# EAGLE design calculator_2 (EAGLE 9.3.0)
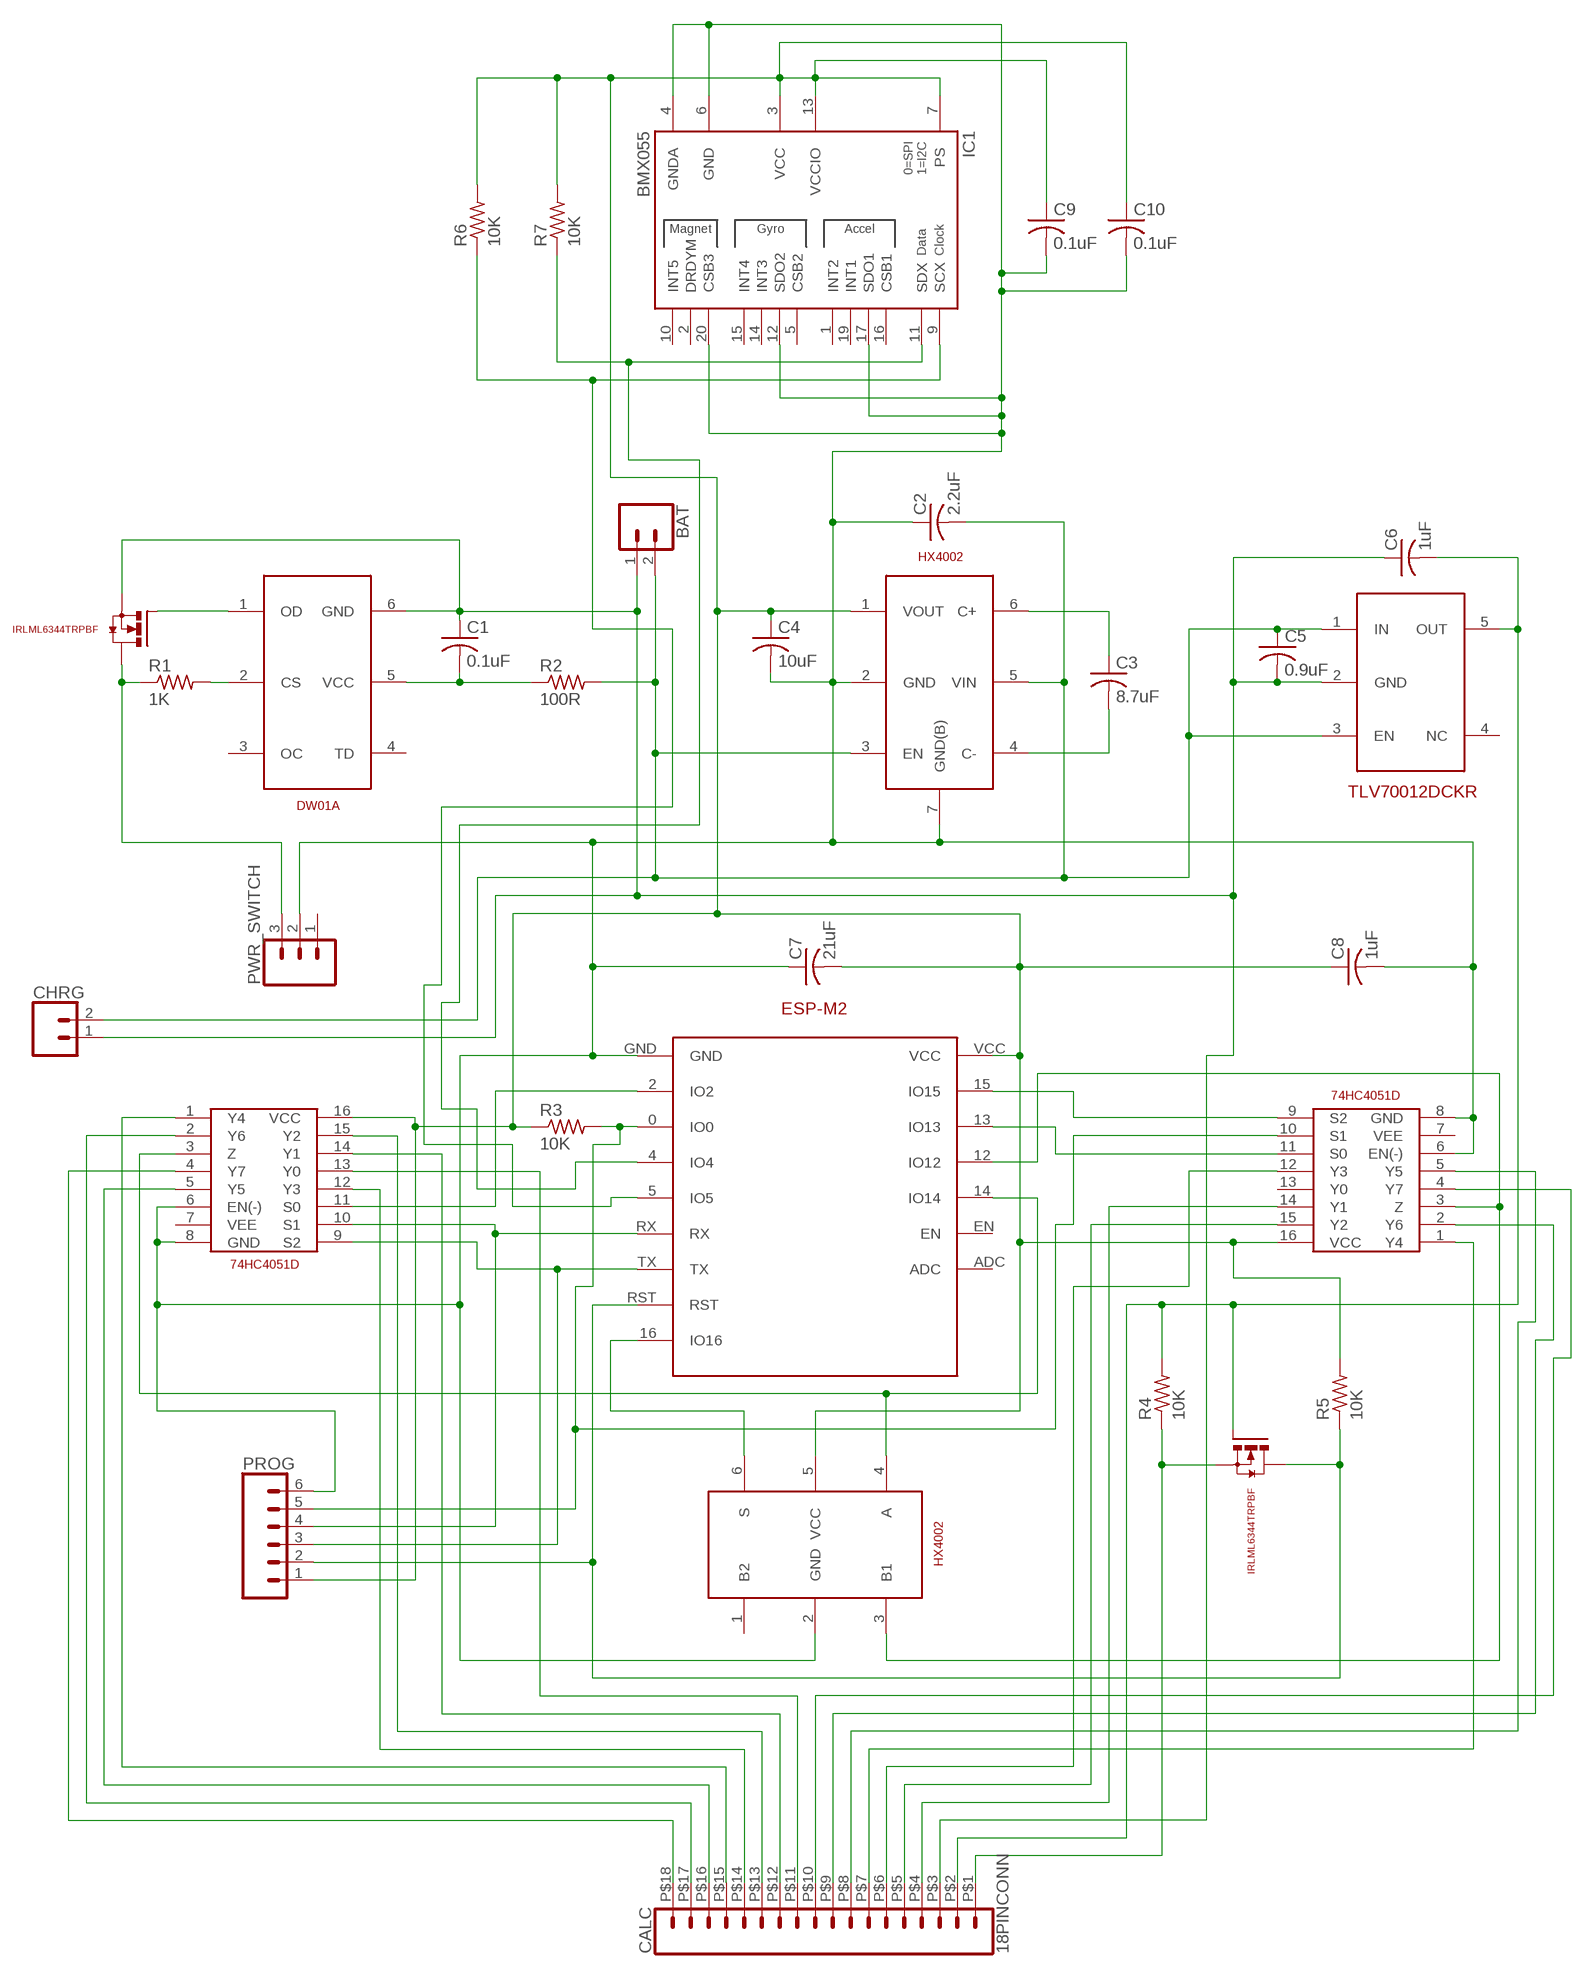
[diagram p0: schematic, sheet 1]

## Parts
BAT  CONN_021X02_NO_SILK  [1X02_NO_SILK]
C1  0.1uF  C-USC0402  [C0402]
C2  2.2uF  C-USC0603  [C0603]
C3  8.7uF  C-USC0402  [C0402]
C4  10uF  C-USC0402  [C0402]
C5  0.9uF  C-USC0402  [C0402]
C6  1uF  C-USC0402  [C0402]
C7  21uF  C-USC0603  [C0603]
C8  1uF  C-USC0603  [C0603]
C9  0.1uF  C-USC0402  [C0402]
C10  0.1uF  C-USC0402  [C0402]
CALC  18PINCONN  [18PINCONN]
CHRG  CONN_021X02_NO_SILK  [1X02_NO_SILK]
ESP-M2  ESP-M2  [ESP-M2]
IC1  BMX055  [BMX055]
IRLML6344  IRLML6344TRPBF6344TRPBF  [SOT-23-3]
PROG  CONN_06NO_SILK_FEMALE_PTH  [1X06_NO_SILK]
PWR_SWITCH  CONN_031X03_NO_SILK  [1X03_NO_SILK]
R1  1K  R-US_R0402  [R0402]
R2  100R  R-US_R0402  [R0402]
R3  10K  R-US_R0402  [R0402]
R4  10K  R-US_R0402  [R0402]
R5  10K  R-US_R0402  [R0402]
R6  10K  R-US_R0402  [R0402]
R7  10K  R-US_R0402  [R0402]
U2  74HC4051  [SOIC-16]
U3  74HC4051  [SOIC-16]
U4  IRLML6344TRPBF6344TRPBF  [SOT-23-3]
U$2  DW01A  [SOT-23-6]
U$3  HX4002  [SOT-23-6(BOTTOM)]
U$4  TLV70012DCKR  [SC70-5]
U$6  SN74LVC1G3157DBVR  [SOT-23-6]

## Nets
GND: C2.1 C4.2 C7.1 C8.2 C9.2 C10.2 ESP-M2.GND IC1.4(GNDA) IC1.6(GND) IC1.12(SDO2) IC1.17(SDO1) IC1.20(CSB3) PROG.6 PWR_SWITCH.2 U2.6(EN(-)) U2.8(GND) U3.6(EN(-)) U3.8(GND) U$3.2(GND) U$3.7(GND(B)) U$6.2(GND)
N$1: IRLML6344.1(G) U$2.1(OD)
N$2: C4.1 C7.2 C8.1 C9.1 C10.1 ESP-M2.VCC IC1.3(VCC) IC1.7(PS) IC1.13(VCCIO) PROG.1 R3.1 R5.2 R6.2 R7.2 U2.16(VCC) U3.16(VCC) U$3.1(VOUT) U$6.5(VCC)
N$3: R1.2 U$2.2(CS)
N$4: BAT.2 C2.2 C5.1 CHRG.2 R2.2 U$3.3(EN) U$3.5(VIN) U$4.1(IN) U$4.3(EN)
N$5: C1.2 R2.1 U$2.5(VCC)
N$6: ESP-M2.0(IO0) PROG.5 R3.2 U3.10(S1)
N$7: C3.1 U$3.6(C+)
N$8: C3.2 U$3.4(C-)
N$9: ESP-M2.13(IO13) U3.11(S0)
N$10: BAT.1 C1.1 C5.2 C6.1 CALC.P$3 CHRG.1 IRLML6344.2(S) U$2.6(GND) U$4.2(GND)
N$11: C6.2 CALC.P$2 R4.2 U4.1(G) U$4.5(OUT)
N$12: ESP-M2.14(IO14) U2.3(Z) U$6.4(A)
N$13: ESP-M2.15(IO15) U3.9(S2)
N$14: ESP-M2.12(IO12) U3.3(Z) U$6.3(B1)
N$15: ESP-M2.TX PROG.3 U2.9(S2)
N$16: ESP-M2.2(IO2) U2.11(S0)
N$17: ESP-M2.RX PROG.4 U2.10(S1)
N$18: ESP-M2.16(IO16) U$6.6(S)
N$19: CALC.P$1 R4.1 U4.2(S)
N$20: IRLML6344.3(D) PWR_SWITCH.3 R1.1
N$21: ESP-M2.4(IO4) IC1.11(SDX) R7.1
N$22: ESP-M2.RST PROG.2 R5.1 U4.3(D)
N$23: CALC.P$4 U3.14(Y1)
N$24: CALC.P$5 U3.15(Y2)
N$25: CALC.P$6 U3.12(Y3)
N$26: CALC.P$7 U3.1(Y4)
N$27: CALC.P$8 U3.5(Y5)
N$28: CALC.P$9 U3.2(Y6)
N$29: CALC.P$10 U3.4(Y7)
N$30: CALC.P$11 U2.13(Y0)
N$31: CALC.P$12 U2.14(Y1)
N$32: CALC.P$13 U2.15(Y2)
N$33: CALC.P$14 U2.12(Y3)
N$34: CALC.P$15 U2.1(Y4)
N$35: CALC.P$16 U2.5(Y5)
N$36: CALC.P$17 U2.2(Y6)
N$37: CALC.P$18 U2.4(Y7)
N$41: ESP-M2.5(IO5) IC1.9(SCX) R6.1
Unconnected: ESP-M2.ADC ESP-M2.EN IC1.1(INT2) IC1.2(DRDYM) IC1.5(CSB2) IC1.10(INT5) IC1.14(INT3) IC1.15(INT4) IC1.16(CSB1) IC1.19(INT1) PWR_SWITCH.1 U2.7(VEE) U3.7(VEE) U3.13(Y0) U$2.3(OC) U$2.4(TD) U$4.4(NC) U$6.1(B2)

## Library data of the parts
BAT CHRG = wifi-calculator-lib:CONN_02: Multi connection point. Often used as Generic Header-pin footprint for 0.1 inch spaced/style header connections
C1-C10 = wifi-calculator-lib:C-US: CAPACITOR, American symbol
CALC = wifi-calculator-lib:18PINCONN
ESP-M2 = wifi-calculator-lib:ESP-M2: ESP8285 Module - M2
IC1 = wifi-calculator-lib:BMX055: Bosch BMX055 Absolute Orientation Sensor (Accelerometer, Gyroscope, Magnetometer)
IRLML6344 U4 = wifi-calculator-lib:IRLML6344TRPBF: N-Channel MOSFET HEXFET® Documentation Datasheet; CATEGORY: Discrete Semiconductor Products; CURRENT-CONTINUOUS_DRAIN: 5A (Ta); DESCRIPTION: MOSFET N-CH 30V 5A SOT23; DOCUMENTATION_LINK: <a href="http://www.irf.com/product-info/datasheets/data/irlml6344pbf.pdf">Datasheet</a>; DOCUMENTATION_URL: http://www.irf.com/product-info/datasheets/data/irlml6344pbf.pdf; DRAIN_TO_SOURCE_VOLTAGE: 30V; FAMILY: FETs - Single; FET_FEATURE: Logic Level Gate; FET_TYPE: MOSFET N-Channel, Metal Oxide; GATE_CHARGE: 6.8nC @ 4.5V; INPUT_CAPACITANCE: 650pF @ 25V; MANUFACTURER: International Rectifier; MOUNTING_TYPE: Surface Mount; PACKAGE: TO-236-3, SC-59, SOT-23-3; PART_NUMBER: IRLML6344TRPBF; POWER-MAX: 1.3W; RDS_ON: 29 mOhm @ 5A, 4.5V; SERIES: HEXFET; SUPPLIER_DEVICE_PACKAGE: SOT-23; SUPPLIER_ITEM_LINK: <a href="http://www.digikey.com/product-detail/en/IRLML6344TRPBF/IRLML6344TRPBFCT-ND/2538168">Details</a>; SUPPLIER_ITEM_NUMBER: IRLML6344TRPBFCT-ND; SUPPLIER_ITEM_URL: http://www.digikey.com/product-detail/en/IRLML6344TRPBF/IRLML6344TRPBFCT-ND/2538168; SUPPLIER_LINK: <a href="http://www.digikey.com">Home Page</a>; SUPPLIER_NAME: Digi-Key; SUPPLIER_URL: http://www.digikey.com; VGS: 1.1V @ 10uA
PROG = wifi-calculator-lib:CONN_06: Multi connection point. Often used as Generic Header-pin footprint for 0.1 inch spaced/style header connections On any of the 0.1 inch spaced packages, you can populate with these: Break Away Headers - Straight (PRT-00116) Break Away Male Headers - Right Angle (PRT-00553) Female Headers (PRT-00115)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; PROD_ID: CONN-08437
PWR_SWITCH = wifi-calculator-lib:CONN_03: Multi connection point. Often used as Generic Header-pin footprint for 0.1 inch spaced/style header connections On any of the 0.1 inch spaced packages, you can populate with these: Break Away Headers - Straight (PRT-00116) Break Away Male Headers - Right Angle (PRT-00553) Female Headers (PRT-00115)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
R1-R7 = wifi-calculator-lib:R-US_: RESISTOR, American symbol
U2 U3 = wifi-calculator-lib:74HC4051: 8 Channel Analog Multiplexer/Demultiplexer
U$2 = wifi-calculator-lib:DW01A: Lithium battery protection IC
U$3 = wifi-calculator-lib:HX4002: 3.3V Output, Buck & Boost Converter
U$4 = wifi-calculator-lib:TLV70012DCKR: 1.2V LDO Voltage Regulator
U$6 = wifi-calculator-lib:SN74LVC1G3157DBVR: Single-Pole Double-Throw Analog Switch

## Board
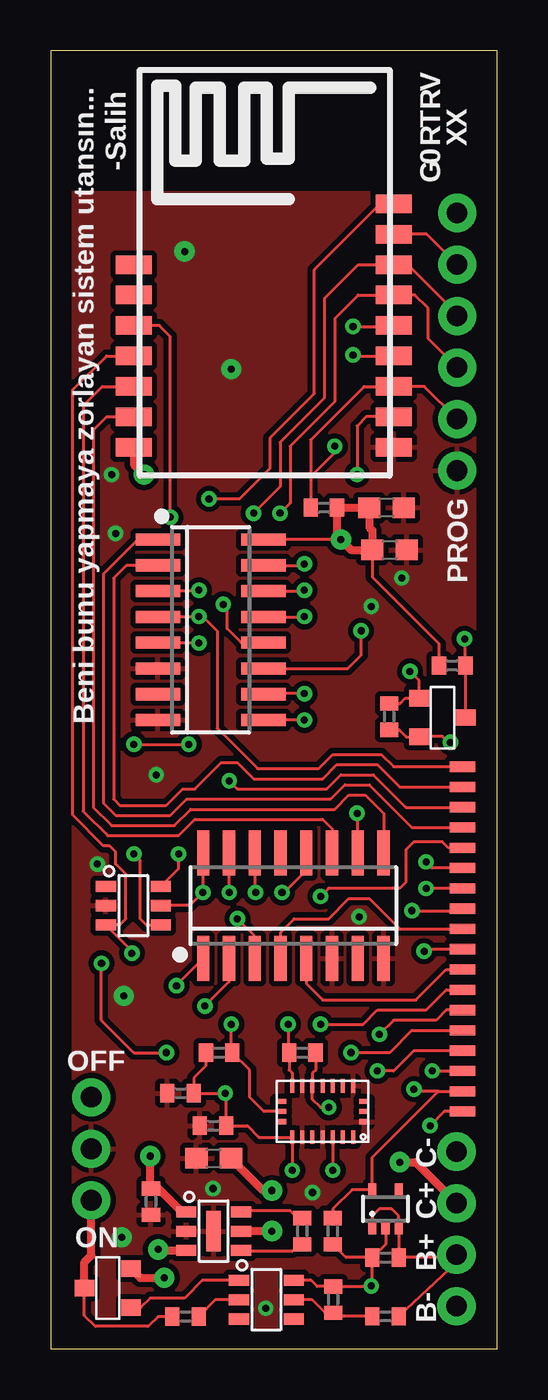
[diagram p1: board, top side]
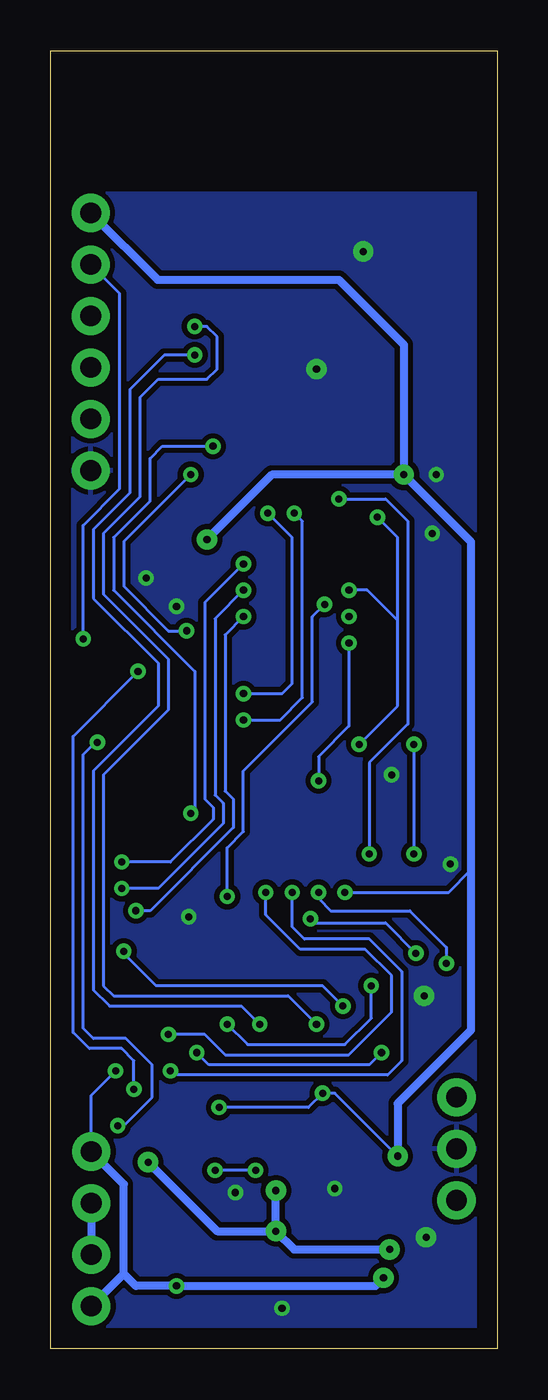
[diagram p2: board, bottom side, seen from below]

Size 22 x 64 mm. Coordinates in mm from the lower left corner, seen from the top.
Outline: 0,0 22,0 22,64 0,64 0,0
Copper layers (1*16): Top 0.035mm / dielectric 1.5mm / Bottom 0.035mm
Design rules "default *": minimum track width 6mil, minimum drill 0.35mm, track to track 6mil, track to pad 6mil, pad to pad 6mil, via to via 6mil, smd to smd 6mil, copper to edge 40mil, drill to drill 6mil, minimum pad ring 10mil, minimum via ring 8mil, stop-mask expansion 4mil, vias tented up to drill 14mil, thermal gap 10mil

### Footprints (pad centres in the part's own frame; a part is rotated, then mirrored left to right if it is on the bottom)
1X02_NO_SILK = drill 1.016 pad 1.88: 1 0,0; 2 2.54,0
C0402 = smd 0.7 x 0.9: 1 -0.65,0; 2 0.65,0
C0603 = smd 1.1 x 1: 1 -0.85,0; 2 0.85,0
18PINCONN = smd 0.5 x 1.27: P$1 -8.5,0; P$2 -7.5,0; P$3 -6.5,0; P$4 -5.5,0; P$5 -4.5,0; P$6 -3.5,0; P$7 -2.5,0; P$8 -1.5,0; P$9 -0.5,0; P$10 0.5,0; P$11 1.5,0; P$12 2.5,0; P$13 3.5,0; P$14 4.5,0; P$15 5.5,0; P$16 6.5,0; P$17 7.5,0; P$18 8.5,0
ESP-M2 = smd 1.778 x 0.914: 0 6,-6.4; 2 6,-7.9; 4 6,-4.9; 5 6,-3.4; 12 -6.8,-4.9; 13 -6.8,-6.4; 14 -6.8,-3.4; 15 -6.8,-7.9; 16 6,2.599; ADC -6.8,-0.4; EN -6.8,-1.9; GND 6,-9.4; RST 6,1.1; RX 6,-1.9; TX 6,-0.4; VCC -6.8,-9.4
BMX055 = smd 0.25 x 0.675: 1 -1.5,1.262; 2 -1,1.262; 3 -0.5,1.262; 4 0,1.262; 5 0.5,1.262; 6 1,1.262; 7 1.5,1.262; 11 1.5,-1.262; 12 1,-1.262; 13 0.5,-1.262; 14 0,-1.262; 15 -0.5,-1.262; 16 -1,-1.262; 17 -1.5,-1.262 | smd 0.55 x 0.25: 8 2.05,0.5; 9 2.05,0; 10 2.05,-0.5; 18 -2.05,-0.5; 19 -2.05,0; 20 -2.05,0.5
SOT-23-3 = smd 0.802 x 0.972: 1 -0.96,-1.15; 2 0.95,-1.15; 3 0,1.15
1X06_NO_SILK = drill 1.016 pad 1.88: 1 0,0; 2 2.54,0; 3 5.08,0; 4 7.62,0; 5 10.16,0; 6 12.7,0
1X03_NO_SILK = drill 1.016 pad 1.88: 1 0,0; 2 2.54,0; 3 5.08,0
R0402 = smd 0.7 x 0.9: 1 -0.65,0; 2 0.65,0
SOIC-16 = smd 2.2 x 0.6: 1 -2.6,4.445; 2 -2.6,3.175; 3 -2.6,1.905; 4 -2.6,0.635; 5 -2.6,-0.635; 6 -2.6,-1.905; 7 -2.6,-3.175; 8 -2.6,-4.445; 9 2.6,-4.445; 10 2.6,-3.175; 11 2.6,-1.905; 12 2.6,-0.635; 13 2.6,0.635; 14 2.6,1.905; 15 2.6,3.175; 16 2.6,4.445
SOT-23-6 = smd 1 x 0.55: 1 -1.35,0.95; 2 -1.35,0; 3 -1.35,-0.95; 4 1.35,-0.95; 5 1.35,0; 6 1.35,0.95
SOT-23-6(BOTTOM) = smd 1 x 0.55: 1 -1.35,0.95; 2 -1.35,0; 3 -1.35,-0.95; 4 1.35,-0.95; 5 1.35,0; 6 1.35,0.95 | smd 0.711 x 1.981: 7 0,0
SC70-5 = smd 0.4 x 0.6: 1 -0.65,-0.95; 2 0,-0.95; 3 0.65,-0.95; 4 0.65,0.95; 5 -0.65,0.95

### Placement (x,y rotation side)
BAT  20,2.1 90 top
C1  13.92,2.42 270 top
C2  8.03,9.4 0 top
C3  12.4,5.8 270 top
C4  4.94,7.25 270 top
C5  16.5,4.5 180 top
C6  13.9,5.8 90 top
C7  16.55,41.47 180 top
C8  16.7,39.39 0 top
C9  8,11 180 top
C10  6.4,12.6 180 top
CALC  20.3,20.2 90 top
CHRG  20,9.72 270 top
ESP-M2  10.9,53.85 0 top
IC1  13.4,11.7 180 top
IRLML6344  2.81,3 90 top
PROG  20.03,56 270 top
PWR_SWITCH  2,12.4 270 top
R1  6.64,1.59 0 top
R2  16.5,1.6 0 top
R3  13.46,41.47 180 top
R4  16.68,31.17 90 top
R5  19.79,33.69 180 top
R6  8.3,14.6 180 top
R7  12.4,14.6 0 top
U2  7.88,35.45 0 top
U3  11.96,21.85 90 top
U4  19.31,31.12 270 top
U$2  10.63,2.42 0 top
U$3  8.03,5.8 0 top
U$4  16.5,6.9 0 top
U$6  4.07,21.85 0 top

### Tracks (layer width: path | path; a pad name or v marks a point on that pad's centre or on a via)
GND  (via drill 0.35, 0.35 pad 1)
  other vias: 8,7.9 17.3,38 15.8,36.6 3.5,5.5 10.6,2 3.6,17.4 15.2,21.3 8.9,48.3 12.9,7.7 2.3,23.9 3.2,40.2 5.2,28.3 6.6,54.1 3,43.1
  pour Bottom (isolate 0.254): 0,57 0,0 22,0 22,57
  pour Top (isolate 0.254): 0,57 0,0 22,0 22,57
N$1
  Top 0.152: U$2.1 7.47,3.37 6.6,2.5 4.9,2.5 4.44,2.04 IRLML6344.1
N$2  (via drill 0.35, 0.35 pad 1)
  Top 0.152: R5.2 19.14,34.75 15.85,38.04 C8.1 | v11.9,8.8 IC1.7 10.26,10.44 9.7,11 C9.1 8.65,12.55 v8.6,12.6 C10.1 7.05,13.35 7.65,13.95 R6.2 | IC1.3 v13.9,8.8 | R7.2 13.05,13.75 12.9,13.6 IC1.13 12.9,12.3 13.3,11.9 v13.7,11.9 | U3.16 7.5,24.43 v7.5,22.5 6.85,21.85 U$6.5 | U2.16 v14.3,39.9
  Top 0.406: U$3.1 6.45,6.75 5.3,7.9 C4.1 4.9,7.94 v4.9,9.5 | ESP-M2.VCC 4.1,43.6 v4.6,43.1 | v14.3,39.9 14.11,40.09 R3.1 C7.2 15.7,40.5 15.85,40.35 C8.1 14.81,39.39 v14.3,39.9
  Bottom 0.152: v11.9,8.8 v13.9,8.8 | v4.9,9.5 8,12.6 v8.6,12.6 9.3,11.9 v13.7,11.9 | v7.5,22.5 2.39,22.5 1.29,23.6
  Bottom 0.406: PROG.1 16.73,52.7 7.8,52.7 4.6,49.5 v4.6,43.1 | v4.6,43.1 11.1,43.1 v14.3,39.9 | v4.6,43.1 1.29,39.79 1.29,23.6 1.29,15.7 4.9,12.09 v4.9,9.5
N$3
  Top 0.152: U$2.2 8.12,2.42 R1.2
N$4  (via drill 0.35 pad 1)
  Top 0.152: R2.2 20,4.26 BAT.2 19.86,4.5 C5.1 U$4.3 17.15,6.55 16.8,6.9 16.2,6.9 15.85,6.55 U$4.1
  Top 0.406: v17.2,9.2 17.98,9.2 CHRG.2 | v10.9,5.8 U$3.5 | v5.3,4.9 5.35,4.85 U$3.3 | v10.9,7.8 10.48,7.8 C2.2
  Bottom 0.406: CHRG.2 BAT.2 | v17.2,9.2 13.8,5.8 v10.9,5.8 | v10.9,5.8 10,4.9 v5.3,4.9 | v10.9,5.8 v10.9,7.8
N$5
  Top 0.152: R2.1 14.09,1.6 C1.2 13.53,1.77 12.88,2.42 U$2.5
N$6  (via drill 0.35)
  Top 0.152: PROG.5 18.42,47.45 ESP-M2.0 15.45,47.45 12.81,44.81 12.81,43 | 12.81,43 R3.2 | 12.81,43 14,44.19 v14,44.5 | v15.1,26.4 15.1,24.48 U3.10
  Bottom 0.152: v15.1,26.4 14.9,26.6 14.9,33.4 18.9,37.4 18.9,40 17.1,41.8 17.1,43.9 16.5,44.5 v14,44.5
N$7
  Top 0.152: C3.1 12.15,6.45 11.8,6.8 9.43,6.8 U$3.6
N$8
  Top 0.152: C3.2 12.25,5.15 11.9,4.8 9.43,4.8 U$3.4
N$9
  Top 0.152: ESP-M2.13 2.55,47.45 1.6,46.5 1.6,26.5 2.8,25.3 6.3,25.3 7.1,26.1 13.4,26.1 13.87,25.64 U3.11
N$10  (via drill 0.35, 0.35 pad 1)
  Top 0.152: U$2.6 12.83,3.37 13.13,3.07 C1.1 15.77,3.07 v15.8,3.1 15.85,3.15 C5.2 | U$4.2 16.5,5.15 C5.2 | C5.2 14.55,4.5 C6.1 | v18.8,13.7 CALC.P$3
  Top 0.406: IRLML6344.2 4.41,3.5 v5.6,3.5
  Bottom 0.152: CHRG.1 20,12.5 v18.8,13.7
  Bottom 0.406: BAT.1 18.4,3.7 | CHRG.1 18.4,8.12 18.4,3.7 | v5.6,3.5 6,3.1 v15.8,3.1 17.8,3.1 18.4,3.7
N$11  (via drill 0.35)
  Top 0.152: C6.2 13.9,6.9 14.85,7.85 U$4.5 15.85,9.45 19.1,12.7 | 19.1,12.7 CALC.P$2 | R4.2 17.22,31.82 17.48,32.08 U4.1 18.16,32.94 v17.7,33.4 | 19.1,12.7 18,12.7 v17.9,12.8
  Bottom 0.152: v17.9,12.8 17.9,14.2 18.5,14.8 20.1,14.8 20.9,15.6 20.9,30.2 v17.7,33.4
N$12  (via drill 0.35)
  Top 0.152: U$6.4 4.7,20.9 4.4,21.2 4.4,24.1 v4.1,24.4 | v4.1,29.8 v6.8,29.8 | v7.3,37.4 7.25,37.35 U2.3 | v5.9,41 5.9,49.9 5.35,50.45 ESP-M2.14
  Bottom 0.152: v4.1,29.8 v4.1,24.4 | v6.8,29.8 4.9,31.7 4.9,35.9 | 4.9,35.9 6.4,37.4 v7.3,37.4 | 4.9,35.9 4.9,40 v5.9,41
N$13
  Top 0.152: U3.9 16.41,26.39 15.5,27.3 14.7,27.3 14,26.6 6.9,26.6 6.1,25.8 3,25.8 2.1,26.7 2.1,45.3 2.75,45.95 ESP-M2.15
N$14  (via drill 0.35)
  Top 0.152: ESP-M2.12 2.75,48.95 1.09,47.29 1.09,26.31 2.6,24.8 2.9,24.8 3.2,24.5 3.2,23.9 3.7,23.4 3.7,21.2 3.4,20.9 U$6.3 4,19.62 v4,19.5 | U3.3 10.05,20.34 v9.2,21.2
  Bottom 0.152: v9.2,21.2 9,21 5.5,21 v4,19.5
N$15  (via drill 0.35)
  Top 0.152: PROG.3 20.03,51.02 17.6,53.45 ESP-M2.TX 15.15,53.45 13.5,51.8 13.5,46.9 11.3,44.7 11.3,42.5 v10,41.2 | v12.5,31 U2.9
  Bottom 0.152: v12.5,31 10.7,31 9.6,32.1 9.6,40.8 v10,41.2
N$16  (via drill 0.35)
  Top 0.152: ESP-M2.2 15.55,45.95 15.1,45.5 v15.1,43.1 | U2.11 14.64,33.55 15.3,34.2 v15.3,35.4
  Bottom 0.152: v15.1,43.1 18.4,39.8 18.4,37.6 16.2,35.4 v15.3,35.4
N$17  (via drill 0.35)
  Top 0.152: PROG.4 18.6,49.81 18.6,51.3 17.95,51.95 ESP-M2.RX 15.15,51.95 14,50.8 14,46.7 11.8,44.5 11.8,41.7 v11.3,41.2 | v12.5,32.3 10.51,32.3 U2.10
  Bottom 0.152: v12.5,32.3 10.6,32.3 10.1,32.8 10.1,40 v11.3,41.2
N$18  (via drill 0.35)
  Top 0.152: ESP-M2.16 16.25,56.45 13,53.2 13,47.1 10.8,44.9 10.8,43.4 9.3,41.9 v7.8,41.9 | U$6.6 6.3,23.68 v6.3,24.4
  Bottom 0.152: v7.8,41.9 5.5,41.9 4.4,40.8 4.4,30.8 6.3,28.9 v6.3,24.4
N$19  (via drill 0.35)
  Top 0.152: R4.1 17.18,30.52 17.53,30.17 U4.2 18.19,30.2 19.3,30.2 19.6,29.9 v19.7,29.9 | CALC.P$1 19.4,11.7 v18.7,11
  Bottom 0.152: v18.7,11 18.4,11 17,12.4 17,14 18.3,15.3 19.9,15.3 20.4,15.8 20.4,29.3 19.8,29.9 v19.7,29.9
N$20
  Top 0.152: R1.1 5.29,1.59 4.8,1.1 2.2,1.1 1.66,1.64 IRLML6344.3
  Top 0.406: IRLML6344.3 1.66,4.26 2,4.6 PWR_SWITCH.3
N$21  (via drill 0.35)
  Top 0.152: IC1.11 11.9,13.6 11.75,13.75 R7.1 11.7,14.65 v11.7,16 | v14.9,49 14.95,48.95 ESP-M2.4
  Bottom 0.152: v14.9,49 16.4,49 18.1,47.3 18.1,42.2 19.9,40.4 19.9,37 16.7,33.8 16.7,31.7 19.9,28.5 19.9,17.7 19.1,16.9 12.6,16.9 v11.7,16
N$22  (via drill 0.35)
  Top 0.152: PROG.2 18.54,54.95 ESP-M2.RST | U4.3 20.46,33.67 R5.1 20.44,34.96 v20.4,35
  Bottom 0.152: v20.4,35 20.4,40.6 18.6,42.4 18.6,52.03 PROG.2
N$23  (via drill 0.35)
  Top 0.152: U3.14 10.05,22.55 v10.1,22.5 | v16.1,13.7 16.9,13.7 17.9,14.7 CALC.P$4
  Bottom 0.152: v10.1,22.5 10.1,20.8 9.5,20.2 6.3,20.2 4.7,18.6 4.7,14.2 5.4,13.5 15.9,13.5 v16.1,13.7
N$24  (via drill 0.35)
  Top 0.152: U3.15 8.79,22.52 v8.8,22.5 | CALC.P$5 17.8,15.7 16.7,14.6 v14.8,14.6 | v5.7,14.6 4.1,14.6 2.5,16.2 v2.5,19
  Bottom 0.152: v8.8,22.5 8.8,22.2 8.2,21.6 4.3,21.6 2.5,19.8 v2.5,19 | v5.7,14.6 6.3,14 14.2,14 v14.8,14.6
N$25  (via drill 0.35)
  Top 0.152: CALC.P$6 19.5,16.7 19,16.2 16.9,16.2 v16.2,15.5 | U3.12 12.6,23.59 11.5,22.5 v11.4,22.5
  Bottom 0.152: v16.2,15.5 14.4,15.5 13.4,14.5 7.3,14.5 5.2,16.6 5.2,18.4 6.5,19.7 9.7,19.7 11.4,21.4 v11.4,22.5
N$26  (via drill 0.35)
  Top 0.152: U3.1 6.2,17.93 v6.2,17.9 | v13.3,16 15.4,16 16.1,16.7 18.5,16.7 19.5,17.7 CALC.P$7
  Bottom 0.152: v13.3,16 12.3,15 7.5,15 6.2,16.3 v6.2,17.9
N$27
  Top 0.152: U3.5 12.6,18 13.4,17.2 18,17.2 19.5,18.7 CALC.P$8
N$28  (via drill 0.35)
  Top 0.152: U3.2 8.79,18.09 v7.6,16.9 | CALC.P$9 18.5,19.7 v18.4,19.6
  Bottom 0.152: v7.6,16.9 8.6,17.9 16.8,17.9 18.4,19.5 v18.4,19.6
N$29
  Top 0.152: U3.4 11.32,20.52 12,21.2 13.7,21.2 14.7,22.2 15.7,22.2 17.2,20.7 CALC.P$10
N$30  (via drill 0.35)
  Top 0.152: U2.13 12.48,36.09 v12.5,36.1 | v17.8,21.6 20.2,21.6 CALC.P$11
  Bottom 0.152: v12.5,36.1 13.4,35.2 13.4,27.5 13,27.1 13,25.7 17.1,21.6 v17.8,21.6
N$31  (via drill 0.35)
  Top 0.152: U2.14 12.46,37.35 v12.5,37.4 | CALC.P$12 v18.5,22.7
  Bottom 0.152: v12.5,37.4 13.9,36 13.9,27.3 13.5,26.9 13.5,25.9 16.7,22.7 v18.5,22.7
N$32  (via drill 0.35)
  Top 0.152: U2.15 12.43,38.62 v12.5,38.7 | CALC.P$13 18.8,23.7 v18.5,24
  Bottom 0.152: v12.5,38.7 14.4,36.8 14.4,27.1 14,26.7 14,26.1 16.1,24 v18.5,24
N$33  (via drill 0.35)
  Top 0.152: CALC.P$14 19.6,24.7 19.3,25 17.9,25 17.5,24.6 17.5,23 17.2,22.7 13.7,22.7 v13.3,22.3 | U2.12 9.38,34.81 8.7,35.5 8.7,36.5 v8.5,36.7
  Bottom 0.152: v13.3,22.3 13.3,24.7 12.5,25.5 12.5,28.5 9.1,31.9 9.1,36.1 v8.5,36.7
N$34
  Top 0.152: U2.1 4.29,39.9 2.6,38.2 2.6,26.9 3.2,26.3 5.9,26.3 6.7,27.1 13.8,27.1 14.5,27.8 15.7,27.8 17.8,25.7 CALC.P$15
N$35  (via drill 0.35)
  Top 0.152: U2.5 7.29,34.81 v7.3,34.8 | v8.8,28 9.2,27.6 13.6,27.6 14.3,28.3 15.9,28.3 17.5,26.7 CALC.P$16
  Bottom 0.152: v7.3,34.8 7.3,30.7 8.8,29.2 v8.8,28
N$36
  Top 0.152: U2.2 3.73,38.62 3.1,38 3.1,27.1 3.4,26.8 5.7,26.8 6.5,27.6 7.1,27.6 8.4,28.9 9.2,28.9 10,28.1 13.4,28.1 14.1,28.8 16.1,28.8 17.2,27.7 CALC.P$17
N$37  (via drill 0.35)
  Top 0.152: U2.4 5.29,36.1 v7.3,36.1 7.5,36.1 8.2,35.4 8.2,30.6 10.2,28.6 13.2,28.6 13.9,29.3 16.3,29.3 16.9,28.7 CALC.P$18
N$41  (via drill 0.35)
  Top 0.152: IC1.9 10.5,11.7 9.8,12.4 9.8,13.75 R6.1 8.9,14.65 v8.9,16 | v14.9,50.4 16.85,50.4 ESP-M2.5
  Bottom 0.152: v8.9,16 10.3,17.4 18.9,17.4 19.4,17.9 19.4,28.3 16.2,31.5 16.2,34 19.4,37.2 19.4,40.2 17.6,42 17.6,46.9 16.7,47.8 14.3,47.8 13.8,48.3 13.8,49.9 14.3,50.4 v14.9,50.4

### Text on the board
tNames: Beni bunu yapmaya zorlayan sistem utansın... | V | R | T | X | R | X | -Salih | 0 | G | OFF | C- | C+ | ON | B+ | B-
